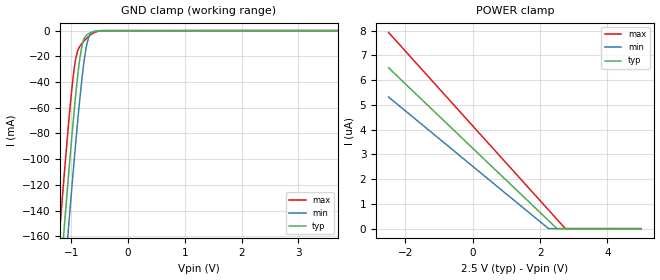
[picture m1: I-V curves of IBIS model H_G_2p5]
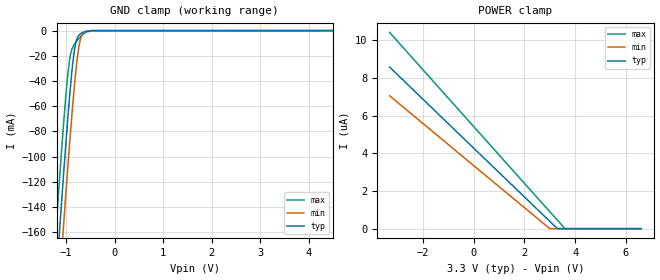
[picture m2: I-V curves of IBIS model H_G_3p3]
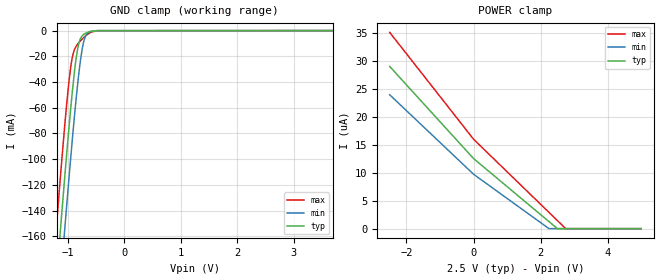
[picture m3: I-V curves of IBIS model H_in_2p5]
| Texas Instruments Incorporated
| 3.3V  LVCMOS High-Performance Clock Buffer
| Signal Rate: 200 kbps
| Marketing part#   Voltage Range   Package-type   #pins/pkg drawing
| cdclvc1104   2.25V - 3.6V   PW   8-pin TSSOP
[IBIS Ver]   4.1
[File name]   cdclvc1104.ibs
[File Rev]   1.0
[Date]   10/26/2010
[Source]   Model built from TISPICE simulations at:
   Texas Instruments Incorporated.
   Analog-eLab, HPA
   12500 TI Blvd
   Dallas, TX -75243
   For Support e-mail: elab_scm_ibis@list.ti.com
[Notes]   Revision History
   Rev 1.0: 08/02/2010
   - Model based on simulations from TIspiceD
   - C_comp values were obtained at 250MHz
   - For all buffers, Ccomp was obtained with the following corners:
   max C_comp was obtained at corner high VCC, low  temperature,
   strong process
   min C_comp was obtained at corner low  VCC, high temperature,
   weak process
   Rev 2.0: 10/26/2010
   - Appl. Eng. requested corrections for Vinh & Vinl
   In H_in_2p5 Vinh should be 1.65V.
   In H_in_3p3 Vinl should be 1.05V.
[Disclaimer] This product is designed as an aid for customers of Texas
   Instruments.
   No warranties, either expressed or implied, with respect
   to this third party software (if any) or with respect to
   its fitness for any particular purpose is claimed by Texas
   Instruments or the author. The software (if any) is provided
   solely on an "as is" basis. The entire risk as to its quality
   and performance is with the customer
[Copyright]   (C)Copyright 2010 Texas Instruments Incorporated.
   All rights reserved.
|   Component cvclvc1104pw
[Component]   cdclvc1104
[Manufacturer]  Texas Instruments Incorporated
[Package]   |8-pin TSSOP package
|   typ   min   max
R_pkg   0.12787   0.01935   0.17743
L_pkg   2.92832nH   1.76351nH   3.62718nH
C_pkg   0.49154pF   0.41852pF   0.53385pF
[Pin] signal_name   model_name   R_pin   L_pin   C_pin
   1   CLKIN   H_in   0.17743  3.62718nH  0.53385pF
   2   1G   H_G   0.16025  2.92096nH  0.49016pF
   3   Y0   H_out   0.16273  2.94718nH  0.49297pF
   4   GND   GND   0.16422  3.50025nH  0.52883pF
   5   Y2   H_out   0.02513  2.35728nH  0.46075pF
   6   VDD   POWER   0.16021  2.92133nH  0.48460pF
   7   Y3   H_out   0.01935  1.76351nH  0.41852pF
   8   Y1   H_out   0.15363  3.38889nH  0.52260pF
[Pin Mapping]pulldown_ref pullup_ref gnd_clamp_ref power_clamp_ref |ext_ref
 1   NC   NC   GNDBUS   PWRBUS   | CLKIN
 2   NC   NC   GNDBUS   PWRBUS   | 1G
 3   GNDBUS   PWRBUS   NC   NC   | Y0
 4   GNDBUS   NC   | GND
 5   GNDBUS   PWRBUS   NC   NC   | Y2
 6   NC   PWRBUS   | VDD
 7   GNDBUS   PWRBUS   NC   NC   | Y3
 8   GNDBUS   PWRBUS   NC   NC   | Y1
[Model Selector] H_G
H_G_2p5   H_G Input model  at 2.5V
H_G_3p3   H_G Input model  at 3.3V
[Model Selector] H_in
H_in_2p5   H_in Input model at 2.5V
H_in_3p3   H_in Input model at 3.3V
[Model Selector] H_out
H_out_2p5   H_out Output model at 2.5V
H_out_3p3   H_out Output model at 3.3V
| Models and submodels in the file (6): H_G_2p5 (Input), H_G_3p3 (Input), H_in_2p5 (Input), H_in_3p3 (Input), H_out_2p5 (Output), H_out_3p3 (Output)
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|   H_G_2p5
[Model]   H_G_2p5
|Signal:   1G
Model_type   Input
Vinl   = 0.85
Vinh   = 1.65
|   typ   min   max
C_comp   910fF   809fF   967fF
[Voltage Range]   2.5   2.25   2.75
[Temperature Range]   25   85   -40
[Power Clamp Reference]   2.5   2.25   2.75
[GND Clamp Reference]   0   0   0
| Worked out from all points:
|   GND clamp passes 1 mA (typ) near -0.62 V on its own axis
[GND Clamp]
|   Voltage   I(typ)   I(min)   I(max)
-2.5V     -968.1mA   -1.007A    -929mA
-1.21V    -199mA     -240.4mA   -156.9mA
-1.15V    -165.5mA   -206.8mA   -123.9mA
-1.12V    -149.1mA   -190.2mA   -107.7mA
-1.064V   -118.8mA   -159.4mA   -78.45mA
-1.045V   -108.9mA   -149.3mA   -69.13mA
-947.5mV  -60.05mA   -98.34mA   -28.07mA
-850mV    -20.81mA   -51.87mA   -12.03mA
-771.2mV  -5.755mA   -21.65mA   -7.739mA
-681.3mV  -1.974mA   -3.841mA   -3.953mA
-463.7mV  -54uA      -32.29uA   -94.42uA
5V        0A         0A         0A
[POWER Clamp]
|   Voltage   I(typ)   I(min)   I(max)
-2.5V     6.5uA      5.321uA    7.929uA
2.251V    325.7nA    0A         752.1nA
2.502V    0A         0A         373.2nA
2.75V     0A         0A         0A
5V        0A         0A         0A
|   H_G_3p3
[Model]   H_G_3p3
|Signal:   1G
Model_type   Input
Vinl   = 1.05
Vinh   = 2.25
|   typ   min   max
C_comp   831.2f   785f   940.5f
[Voltage Range]   3.3   3   3.6
[Temperature Range]   25   85   -40
[Power Clamp Reference]   3.3   3   3.6
[GND Clamp Reference]   0   0   0
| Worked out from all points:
|   GND clamp passes 1 mA (typ) near -0.62 V on its own axis
[GND Clamp]
|   Voltage   I(typ)   I(min)   I(max)
-3.3V     -1.461A    -1.498A    -1.424A
-1.221V   -205.1mA   -246.6mA   -163.1mA
-1.206V   -196.8mA   -238.2mA   -154.8mA
-1.137V   -158.3mA   -199.5mA   -116.7mA
-1.063V   -118.2mA   -158.8mA   -77.87mA
-993.3mV  -82.31mA   -121.9mA   -45.27mA
-933.9mV  -53.76mA   -91.51mA   -24.11mA
-834.9mV  -16.5mA    -45.37mA   -11.07mA
-790.3mV  -7.806mA   -28.02mA   -8.666mA
-730.9mV  -3.374mA   -11.05mA   -5.922mA
-632mV    -1.127mA   -1.236mA   -2.355mA
6.6V      0A         0A         0A
[POWER Clamp]
|   Voltage   I(typ)   I(min)   I(max)
-3.3V     8.58uA     7.058uA    10.42uA
3.001V    391.5nA    0A         903.2nA
3.303V    0A         0A         447.8nA
3.6V      0A         0A         0A
6.6V      0A         0A         0A
|   H_in_2p5
[Model]   H_in_2p5
|Signal:   CLK_IN
Model_type   Input
Vinl   = 0.85
Vinh   = 1.65
|   typ   min   max
C_comp   0.943pF   0.765pF   1.207pF
[Voltage Range]   2.5   2.25   2.75
[Temperature Range]   25   85   -40
[Power Clamp Reference]   2.5   2.25   2.75
[GND Clamp Reference]   0   0   0
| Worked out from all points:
|   GND clamp passes 1 mA (typ) near -0.62 V on its own axis
[GND Clamp]
|   Voltage   I(typ)   I(min)   I(max)
-2.5V     -968.1mA   -1.007A    -929mA
-1.21V    -199mA     -240.4mA   -156.9mA
-1.15V    -165.6mA   -206.8mA   -123.9mA
-1.12V    -149.1mA   -190.2mA   -107.7mA
-1.064V   -118.8mA   -159.4mA   -78.47mA
-1.045V   -108.9mA   -149.3mA   -69.14mA
-947.5mV  -60.06mA   -98.34mA   -28.08mA
-850mV    -20.82mA   -51.87mA   -12.04mA
-771.2mV  -5.763mA   -21.66mA   -7.749mA
-681.3mV  -1.981mA   -3.847mA   -3.963mA
-463.7mV  -60.38uA   -37.46uA   -102.3uA
5V        0A         0A         0A
[POWER Clamp]
|   Voltage   I(typ)   I(min)   I(max)
-2.5V     29.05uA    23.98uA    35.15uA
1.25mV    12.55uA    9.742uA    16.01uA
2.251V    1.261uA    0A         2.905uA
2.502V    0A         0A         1.442uA
2.75V     0A         0A         0A
5V        0A         0A         0A
